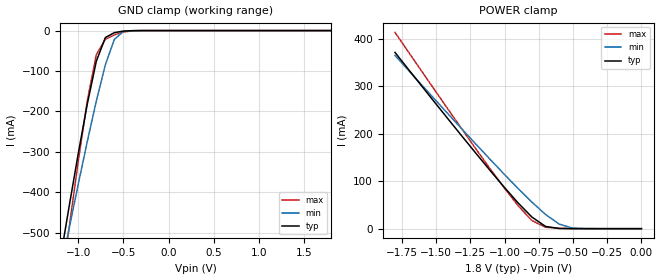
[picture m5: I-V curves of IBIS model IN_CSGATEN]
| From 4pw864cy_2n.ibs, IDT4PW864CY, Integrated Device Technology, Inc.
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|   Model IN_CSGATEN
[Model]   IN_CSGATEN
Model_type   Input
Vinl =  0.000V
Vinh =  1.80000V
C_comp   1.750000pF   1.75000pF   1.75000pF
[Temperature Range]   25.00000   0.11000k   0.000
[Voltage Range]   1.80000V   1.70000V   1.90000V
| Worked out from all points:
|   GND clamp passes 1 mA (typ) near -0.48 V on its own axis
|   POWER clamp passes 1 mA (typ) near -0.61 V on its own axis
[GND_clamp]
| voltage   I(typ)   I(min)   I(max)
-1.8V     -1.393A    -1.281A    -1.7A
-1.2V     -567.6mA   -599.8mA   -654.6mA
-1.1V     -434.5mA   -489.3mA   -486.7mA
-1V       -304.9mA   -380.6mA   -324.4mA
-900mV    -182.1mA   -274.9mA   -174mA
-800mV    -75.99mA   -174.5mA   -59.62mA
-700mV    -17.34mA   -84.78mA   -21.72mA
-600mV    -5.059mA   -21.72mA   -10.57mA
-500mV    -1.248mA   -2.195mA   -3.453mA
-300mV    -24.99uA   -16.39uA   -91.03uA
1.8V      2.188nA    17.19nA    1.672nA
[POWER_clamp]
| voltage   I(typ)   I(min)   I(max)
-1.8V     371.6mA    365.3mA    413.8mA
-1.4V     226.9mA    238.1mA    246.6mA
-1.1V     120.9mA    144.6mA    124.3mA
-900mV    53.99mA    84.46mA    48.22mA
-800mV    24.48mA    55.97mA    17.07mA
-700mV    4.619mA    29.87mA    2.867mA
-600mV    374.6uA    9.474mA    727.9uA
-500mV    44.79uA    1.038mA    142.1uA
0V        2.188nA    1.932nA    1.881nA
